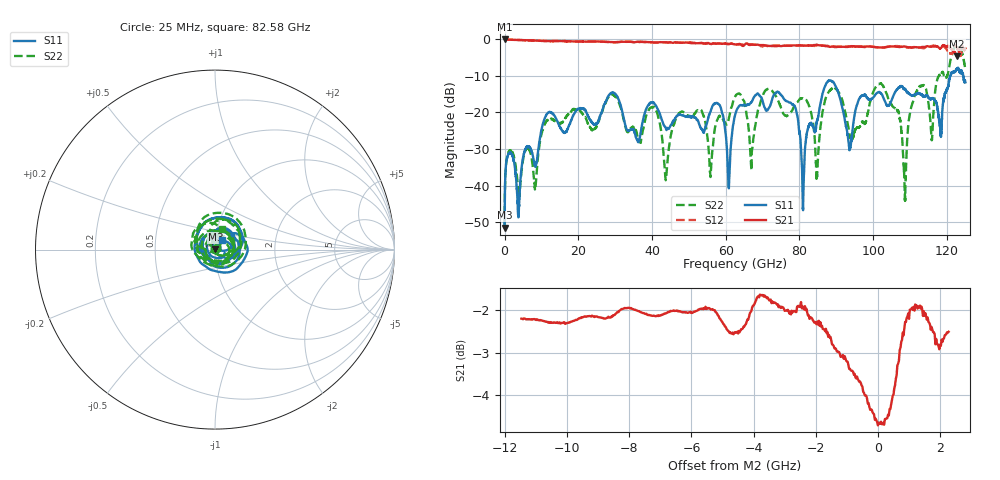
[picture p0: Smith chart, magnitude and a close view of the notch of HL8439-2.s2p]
! 3/1/2024 1:19:42 PM
! H:\PROTOTYPE_DATA\AMOTECH 110G\GROUND WITH BIGGER HOLE-2.S2P
! CHANNEL.1
! TR.MEASUREMENT
! CORRECTED.DATA
! RF.CORRECTION: FULL.TWO.PORT.CAL.PORT.1.2
! AVERAGING: 1 PointByPoint
! IF.BANDWIDTH: 1KHZ
! SWEEPTYPE:  FREQ.SWEEP(Linear)
! Reference Plane Port Info
! PORT:  PORT1  PORT2
! DISTANCE:  0  m  0  m
! TIME:  0  s  0  s
! PHASE.OFFSET:  0 °  0 °
! LOSS:  0  dB  0  dB
! REF.LOSS:  0  dB  0  dB
! REF.FREQ:  0  Hz  0  Hz
! Power Info
! POWER:  -10  dBm  -10  dBm
! EFF.POWER:  -10  dBm  -10  dBm
! POWER(>54G):  -10  dBm  -10  dBm
! EFF.POWER(>54G):  -10  dBm  -10  dBm
! SOURCE.ATTEN:  0  dB  0  dB
! TEST.ATTEN:  0  dB  0  dB
# GHZ S RI R 50.0
! FREQ.GHZ  S11RE  S11IM  S21RE  S21IM  S12RE  S12IM  S22RE  S22IM
!; PortSelection: Port_12
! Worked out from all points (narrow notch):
!   5000 points, 25 MHz to 125 GHz, reference 50 ohm
!   highest |S21| = -0.02 dB at 25 MHz (marker M1); lowest = -4.7 dB at 122.7 GHz (marker M2)
!   notch at M2: 3.4 dB deep, 1.92 GHz wide at half that depth
!   lowest |S11| = -51.4 dB at 25 MHz (marker M3), VSWR 1.01, Z = 50.2 + j0.197 ohm
!   |S11| at or under -10 dB: start of sweep to 121 GHz; 124.4122 GHz to end of sweep
!   |S22| runs from -51.3 to -1.8 dB; largest |S21 - S12| = 0.21
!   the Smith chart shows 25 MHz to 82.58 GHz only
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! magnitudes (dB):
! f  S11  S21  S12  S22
! 25 MHz  -51.4  0.0  0.0  -51.3
! 1.375 GHz  -31.0  -0.2  -0.2  -30.5
! 3.775 GHz  -48.6  -0.3  -0.3  -42.4
! 11.5 GHz  -20.4  -0.5  -0.5  -22.2
! 20.88 GHz  -18.9  -0.7  -0.7  -20.0
! 41.7 GHz  -19.4  -0.9  -0.9  -21.3
! 43.73 GHz  -24.2  -0.9  -0.9  -38.5
! 48.02 GHz  -20.8  -1.0  -1.0  -19.8
! 55.92 GHz  -19.7  -1.4  -1.2  -36.7
! 60.83 GHz  -40.6  -1.3  -1.4  -21.6
! 62.52 GHz  -20.7  -1.4  -1.4  -15.7
! 67 GHz  -17.2  -1.6  -1.4  -35.8
! 71.25 GHz  -19.4  -1.8  -1.9  -13.7
! 78.53 GHz  -18.1  -1.7  -1.8  -18.3
! 80.95 GHz  -46.0  -1.7  -1.8  -16.2
! 83.35 GHz  -23.4  -1.8  -1.7  -20.9
! 104.2 GHz  -18.1  -2.1  -2.1  -16.7
! 108.6 GHz  -13.7  -2.1  -2.3  -41.4
! 111.7 GHz  -15.1  -2.2  -2.3  -14.4
! 115.8 GHz  -16.3  -2.1  -1.9  -27.6
! 122.7 GHz  -8.3  -4.7  -2.5  -2.3
! 125 GHz  -11.8  -2.5  -2.8  -8.3
